(* Logix 5000 DataType export R203_Seneca_InData; software revision 35.00 *)

TYPE R203_Seneca_InData :   // User Define Measure Data Type for Seneca R203-E Advanced Power Meter Device
STRUCT
   VL1L2 : REAL;
   VL2L3 : REAL;
   VL3L1 : REAL;
   VL1N : REAL;
   VL2N : REAL;
   VL3N : REAL;
   IL1 : REAL;
   IL2 : REAL;
   IL3 : REAL;
   IN : REAL;
   ACTIVE_POWER_L1 : REAL;
   ACTIVE_POWER_L2 : REAL;
   ACTIVE_POWER_L3 : REAL;
   REACTIVE_POWER_L1 : REAL;
   REACTIVE_POWER_L2 : REAL;
   REACTIVE_POWER_L3 : REAL;
   APPARENT_POWER_L1 : REAL;
   APPARENT_POWER_L2 : REAL;
   APPARENT_POWER_L3 : REAL;
   TOTAL_ACTIVE_POWER : REAL;
   TOTAL_REACTIVE_POWER : REAL;
   TOTAL_APPARENT_POWER : REAL;
   ANGLE_VI_L1 : REAL;
   ANGLE_VI_L2 : REAL;
   ANGLE_VI_L3 : REAL;
   ANGLE_VI_L1_L2 : REAL;
   ANGLE_VI_L2_L3 : REAL;
   ANGLE_VI_L3_L1 : REAL;
   POWER_FACTOR_L1 : REAL;
   POWER_FACTOR_L2 : REAL;
   POWER_FACTOR_L3 : REAL;
   POWER_FACTOR_TOTAL : REAL;
   FREQUENCY_L1 : REAL;
   FREQUENCY_L2 : REAL;
   FREQUENCY_L3 : REAL;
   PERIOD_L1 : REAL;
   PERIOD_L2 : REAL;
   PERIOD_L3 : REAL;
   THD_V_L1 : REAL;
   THD_V_L2 : REAL;
   THD_V_L3 : REAL;
   THD_I_L1 : REAL;
   THD_I_L2 : REAL;
   THD_I_L3 : REAL;
   AVG_V_L1 : REAL;
   AVG_V_L2 : REAL;
   AVG_V_L3 : REAL;
   AVG_I_L1 : REAL;
   AVG_I_L2 : REAL;
   AVG_I_L3 : REAL;
   AVG_ACTIVE_POWER_3PH : REAL;
   AVG_REACTIVE_POWER_3PH : REAL;
   AVG_APPARENT_POWER_3PH : REAL;
   MIN_V_L1 : REAL;
   MIN_V_L2 : REAL;
   MIN_V_L3 : REAL;
   MIN_I_L1 : REAL;
   MIN_I_L2 : REAL;
   MIN_I_L3 : REAL;
   MIN_ACTIVE_POWER_3PH : REAL;
   MIN_REACTIVE_POWER_3PH : REAL;
   MIN_APPARENT_POWER_3PH : REAL;
   MAX_V_L1 : REAL;
   MAX_V_L2 : REAL;
   MAX_V_L3 : REAL;
   MAX_I_L1 : REAL;
   MAX_I_L2 : REAL;
   MAX_I_L3 : REAL;
   MAX_ACTIVE_POWER_3PH : REAL;
   MAX_REACTIVE_POWER_3PH : REAL;
   MAX_APPARENT_POWER_3PH : REAL;
   ENERGY_ACTIVE_POS_Q1Q4_L1 : REAL;
   ENERGY_ACTIVE_POS_Q1Q4_L2 : REAL;
   ENERGY_ACTIVE_POS_Q1Q4_L3 : REAL;
   ENERGY_ACTIVE_NEG_Q2Q3_L1 : REAL;
   ENERGY_ACTIVE_NEG_Q2Q3_L2 : REAL;
   ENERGY_ACTIVE_NEG_Q2Q3_L3 : REAL;
   ENERGY_ACTIVE_TOTAL_L1 : REAL;
   ENERGY_ACTIVE_TOTAL_L2 : REAL;
   ENERGY_ACTIVE_TOTAL_L3 : REAL;
   ENERGY_ACTIVE_3PH_POS_Q1Q4 : REAL;
   ENERGY_ACTIVE_3PH_NEG_Q2Q3 : REAL;
   ENERGY_ACTIVE_TOTAL_3PH : REAL;
   ENERGY_REACTIVE_POS_Q1Q2_L1 : REAL;
   ENERGY_REACTIVE_POS_Q1Q2_L2 : REAL;
   ENERGY_REACTIVE_POS_Q1Q2_L3 : REAL;
   ENERGY_ACTIVE_3PH_POS_Q1Q2 : REAL;
   ENERGY_REACTIVE_NEG_Q3Q4_L1 : REAL;
   ENERGY_REACTIVE_NEG_Q3Q4_L2 : REAL;
   ENERGY_REACTIVE_NEG_Q3Q4_L3 : REAL;
   ENERGY_ACTIVE_3PH_NEG_Q3Q4 : REAL;
   ENERGY_REACTIVE_POS_Q1_L1 : REAL;
   ENERGY_REACTIVE_POS_Q1_L2 : REAL;
   ENERGY_REACTIVE_POS_Q1_L3 : REAL;
   ENERGY_REACTIVE_NEG_Q2_L1 : REAL;
   ENERGY_REACTIVE_NEG_Q2_L2 : REAL;
   ENERGY_REACTIVE_NEG_Q2_L3 : REAL;
   ENERGY_REACTIVE_POS_Q3_L1 : REAL;
   ENERGY_REACTIVE_POS_Q3_L2 : REAL;
   ENERGY_REACTIVE_POS_Q3_L3 : REAL;
   ENERGY_REACTIVE_NEG_Q4_L1 : REAL;
   ENERGY_REACTIVE_NEG_Q4_L2 : REAL;
   ENERGY_REACTIVE_NEG_Q4_L3 : REAL;
   ENERGY_REACTIVE_TOTAL_L1 : REAL;
   ENERGY_REACTIVE_TOTAL_L2 : REAL;
   ENERGY_REACTIVE_TOTAL_L3 : REAL;
   ENERGY_REACTIVE_TOTAL_3PH : REAL;
   ENERGY_APPARENT_TOTAL_L1 : REAL;
   ENERGY_APPARENT_TOTAL_L2 : REAL;
   ENERGY_APPARENT_TOTAL_L3 : REAL;
   ENERGY_APPARENT_TOTAL_3PH : REAL;
   ENERGY_REACTIVE_ABSORBED_POS_TOTAL_3PH : REAL;
   ENERGY_REACTIVE_ABSORBED_NEG_TOTAL_3PH : REAL;
   ENERGY_REACTIVE_DELIVERED_POS_TOTAL_3PH : REAL;
   ENERGY_REACTIVE_DELIVERED_NEG_TOTAL_3PH : REAL;
   COUNT1 : UDINT;
   COUNT2 : UDINT;
   DIN1 : BOOL;
   DIN2 : BOOL;
   UNUSED1 : BOOL;
   UNUSED2 : BOOL;
   UNUSED3 : BOOL;
   UNUSED4 : BOOL;
   UNUSED5 : BOOL;
   UNUSED6 : BOOL;
   CYCLE_PHASE_ERR : BOOL;
   NOT_USED : BOOL;
   CURR_ERR_L1 : BOOL;
   CURR_ERR_L2 : BOOL;
   CURR_ERR_L3 : BOOL;
   ERR_L1 : BOOL;
   ERR_L2 : BOOL;
   ERR_L3 : BOOL;
END_STRUCT
END_TYPE
